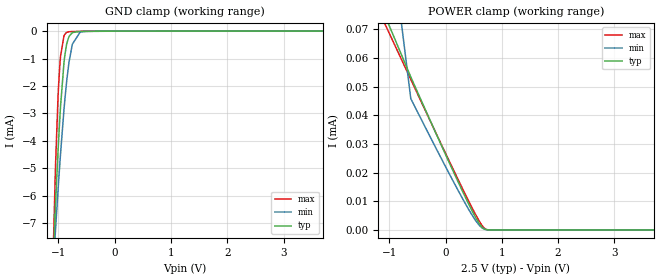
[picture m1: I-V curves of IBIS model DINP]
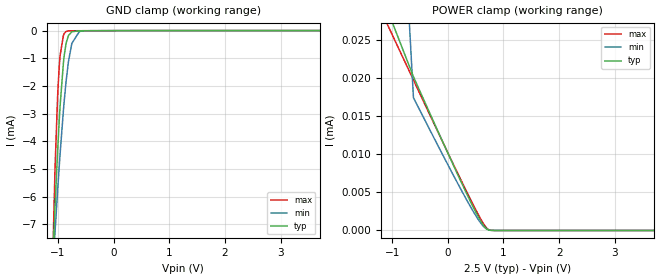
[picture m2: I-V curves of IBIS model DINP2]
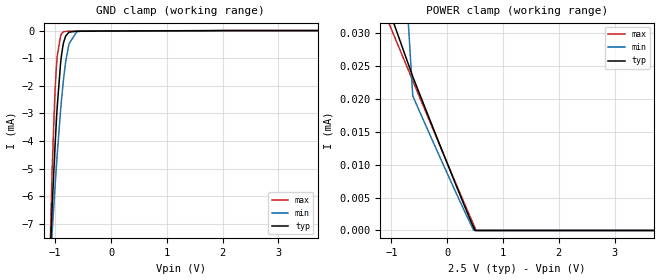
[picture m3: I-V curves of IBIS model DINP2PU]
| Texas Instruments Incorporated
| Wideband Frequency Multiplier/Buffer/Divider
| Marketing part#   Voltage Range   Package-type   #pins/pkg drawing
| LMX1906PAP   2.4V - 2.6V   HTQFP   64
[IBIS Ver]   4.1
[File name]   lmx1906.ibs
[File Rev]   1.0
[Date]   12/15/2023
[Source]   Model built from spectre simulations at:
   Texas Instruments Incorporated.
   Analog-eLab, HPA
   12500 TI Blvd
   Dallas, TX -75243
   For Support e-mail: elab_ibis@list.ti.com
[Notes]   Revision History
   Rev 1.0: 12/15/2023
   | - Initial version of the model
		| - Model generated from simulations in TISPICE/SPECTRE
		| - C_comp although listed in numerical order of value are
		| obtained from varying PVT conditions. For PVT conditions for
		| each specific value refer the buffer description under
		| respective [Model]. IBIS model user is responsible for using
		| appropriate C_comp to simulate for Signal Integrity.
		| - Warnings regarding combined Non-monotonicity of various models have been
		| reviewed and considered minor and can be ignored.
[Disclaimer]  This model is designed as an aid for customers of Texas Instruments
 TI and its licensors and suppliers make no warranties, either expressed
 or implied, with respect to this  model, including the warranties of
 merchantability or fitness for a particular purpose.
 The model is provided solely on an "as is" basis. The entire risk as to
 its quality and performance is with the customer.
[Copyright] (C)Copyright 2022 Texas Instruments Incorporated.
   All rights reserved.
[Component]   LMX1906PAP
[Manufacturer]  Texas Instruments Incorporated
[Package]   | 64 HTQFP package
|   typ   min   max
R_pkg   0.1725   0.1129   0.2855
L_pkg   2.714n   2.2186n   3.5183n
C_pkg   0.361p   0.314p   0.430p
[Pin]   signal_name   model_name   R_pin   L_pin   C_pin
1		MUXOUT			MUXOUT   0.2855	3.3842n	0.3415p
2		CE   DINP2PU   0.2536	3.3372n	0.3506p
3		SYSREFREQ_P		SYSREFREQ			0.1427	2.5185n	0.4062p
4		SYSREFREQ_N		SYSREFREQ			0.1446	2.4677n	0.4029p
5		VCC_CLKIN		POWER   0.1444	2.4377n	0.4011p
6		GND   GND   0.1465	2.5401n	0.4093p
7		CLKIN_P			CLKIN   0.1378	2.5513n	0.3934p
8		CLKIN_N			CLKIN   0.1335	2.5574n	0.3858p
9		GND   GND   0.1276	2.5225n	0.3644p
10		PWRSEL0			DINP2   0.2286	3.1682n	0.3091p
11		PWRSEL1			DINP2   0.2255	3.1183n	0.3252p
12		PWRSEL2			DINP2   0.2354	3.0653n	0.3145p
13		NC   NC   NA		NA		0.1876p
14		SCK   DINP   0.2413	3.2102n	0.3359p
15		SDI   DINP   0.2507	3.3356n	0.3545p
16		CSB   DINP   0.2811	3.4095n	0.3313p
17		CAL   DINP2PD   0.2609	3.2904n	0.3177p
18		SYSREFOUT0_N	SYSREFOUT			0.1338	2.4339n	0.4106p
19		SYSREFOUT0_P	SYSREFOUT			0.1337	2.346n	0.4077p
20		VCC01			POWER   0.125	2.3265n	0.3695p
21		GND   GND   0.1219	2.3195n	0.3653p
22		CLKOUT0_N		CLKOUT   0.1183	2.2631n	0.3573p
23		CLKOUT0_P		CLKOUT   0.1158	2.2412n	0.3551p
24		GND   GND   0.1129	2.2186n	0.3405p
25		CLK0_EN			DINP2PU   0.2001	2.7673n	0.2962p
26		CLK1_EN			DINP2PU   0.2022	2.7921n	0.2955p
27		VCC01			POWER   0.1158	2.2646n	0.3559p
28		GND   GND   0.1214	2.3129n	0.3748p
29		CLKOUT1_N		CLKOUT   0.1258	2.3939n	0.3804p
30		CLKOUT1_P		CLKOUT   0.13	2.4419n	0.3917p
31		GND   GND   0.1391	2.5338n	0.4304p
32		VBIAS01			NC   0.1511	2.6436n	0.3713p
33		SYSREFOUT1_N	SYSREFOUT			0.1629	2.6698n	0.3981p
34		SYSREFOUT1_P	SYSREFOUT			0.1536	2.6121n	0.4289p
35		DIVSEL2			DINP2   0.2536	3.4411n	0.3494p
36		DIVSEL1			DINP2   0.2393	3.3209n	0.3437p
37		DIVSEL0			DINP2   0.23	3.2291n	0.3392p
38		LOGISYSREFOUT_N	LOGICOUT			0.2284	3.2104n	0.3111p
39		LOGISYSREFOUT_P	LOGICOUT			0.2274	3.1382n	0.3282p
40		VCC_LOGICLK		POWER   0.1269	2.4538n	0.3782p
41		GND   GND   0.133	2.3535n	0.3903p
42		LOGICLKOUT_N	LOGICOUT			0.2374	2.9999n	0.3282p
43		LOGICLKOUT_P	LOGICOUT			0.2299	3.1823n	0.3066p
44		LOGIC_EN		DINP2PU   0.2321	3.2611n	0.3316p
45		MUXSEL1			DINP2   0.2423	3.3821n	0.3494p
46		MUXSEL0			DINP2   0.2574	3.5183n	0.3459p
47		SYSREFOUT2_N	SYSREFOUT			0.1535	2.6397n	0.4253p
48		SYSREFOUT2_P	SYSREFOUT			0.1637	2.6631n	0.4082p
49		VBIAS23			NC   0.1492	2.6652n	0.3821p
50		GND   GND   0.1387	2.5423n	0.4206p
51		CLKOUT2_N		CLKOUT   0.1303	2.4448n	0.3945p
52		CLKOUT2_P		CLKOUT   0.1259	2.395n	0.3887p
53		GND   GND   0.1217	2.315n	0.3737p
54		VCC23			POWER   0.116	2.2652n	0.373p
55		CLK2_EN			DINP2PU   0.2023	2.7925n	0.3032p
56		CLK3_EN			DINP2PU   0.2001	2.768n	0.2971p
57		GND   GND   0.1129	2.2196n	0.3488p
58		CLKOUT3_N		CLKOUT   0.1161	2.2426n	0.3563p
59		CLKOUT3_P		CLKOUT   0.1182	2.2641n	0.3735p
60		GND   GND   0.1225	2.3228n	0.3619p
61		VCC23			POWER   0.1255	2.3319n	0.3762p
62		SYSREFOUT3_N	SYSREFOUT			0.1341	2.3637n	0.4173p
63		SYSREFOUT3_P	SYSREFOUT			0.1341	2.441n	0.421p
64		SYSREF_EN		DINP2PU   0.2593	3.3219n	0.3135p
[Diff pin]  inv_pin  vdiff  tdelay_typ  tdelay_min  tdelay_max
  3   4   NA   NA   NA   NA
  7   8   NA   NA   NA   NA
 19   18   NA   0.0s   0.0s   0.0s
 23   22   NA   0.0s   0.0s   0.0s
 30   29   NA   0.0s   0.0s   0.0s
 34   33   NA   0.0s   0.0s   0.0s
 39   38   NA   0.0s   0.0s   0.0s
 43   42   NA   0.0s   0.0s   0.0s
 48   47   NA   0.0s   0.0s   0.0s
 52   51   NA   0.0s   0.0s   0.0s
 59   58   NA   0.0s   0.0s   0.0s
 63   62   NA   0.0s   0.0s   0.0s
| Models and submodels in the file (10): DINP (Input), DINP2 (Input), DINP2PU (Input), DINP2PD (Input), MUXOUT (Output), CLKIN (Input), SYSREFREQ (Input), CLKOUT (Output), SYSREFOUT (Output), LOGICOUT (Output)
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|   Model DINP
[Model]   DINP
Model_type   Input
Vinl = 0.4
Vinh = 1.4
|   typ   min   max
C_comp   0.0195pF   0.0186pF   0.0315pF
[Voltage Range]   2.5   2.4   2.6
[Temperature Range]   27   105   -40
[Power Clamp Reference]   2.5   2.4   2.6
[GND Clamp Reference]   0   0   0
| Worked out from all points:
|   GND clamp passes 1 mA (typ) near -0.89 V on its own axis
|   POWER clamp passes 1 mA (typ) near -1.77 V on its own axis
[GND Clamp]
|   Voltage   I(typ)   I(min)   I(max)
-2.5V     -99.67mA   -67.42mA   -181.3mA
-1.113V   -9.277mA   -9.317mA   -9.589mA
-1.052V   -6.327mA   -7.259mA   -4.916mA
-1.008V   -4.376mA   -5.809mA   -2.402mA
-977.5mV  -3.241mA   -4.898mA   -1.299mA
-962.5mV  -2.733mA   -4.463mA   -914.2uA
-902.5mV  -1.168mA   -2.88mA    -182.1uA
-850mV    -435.4uA   -1.755mA   -43.32uA
-812.5mV  -195.5uA   -1.133mA   -23.19uA
-752.5mV  -53.81uA   -476.9uA   -16.37uA
-572.5mV  -11.42uA   -23.03uA   -8.659uA
5V        0A         0A         0A
[POWER Clamp]
|   Voltage   I(typ)   I(min)   I(max)
-2.5V     13.01mA    14.14mA    11.88mA
-1.337V   87.06uA    159.9uA    82.89uA
-617.5mV  53.41uA    45.83uA    52.55uA
-47.5mV   28.4uA     23.9uA     28.74uA
327.5mV   12.45uA    10.06uA    13.4uA
545mV     3.985uA    2.992uA    4.984uA
605mV     2.064uA    1.51uA     2.9uA
680mV     464.7nA    375.9nA    816.5nA
725mV     113.8nA    119.2nA    188.1nA
807.5mV   4.801nA    11.39nA    3.57nA
5V        0A         0A         0A
|   Model DINP2
[Model]   DINP2
Model_type   Input
Vinl = 0.4
Vinh = 1.4
|   typ   min   max
C_comp   0.0195pF   0.0186pF   0.0315pF
[Voltage Range]   2.5   2.4   2.6
[Temperature Range]   27   105   -40
[Power Clamp Reference]   2.5   2.4   2.6
[GND Clamp Reference]   0   0   0
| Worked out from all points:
|   GND clamp passes 1 mA (typ) near -0.89 V on its own axis
|   POWER clamp passes 1 mA (typ) near -1.77 V on its own axis
[GND Clamp]
|   Voltage   I(typ)   I(min)   I(max)
-2.5V     -99.57mA   -67.32mA   -181.2mA
-1.113V   -9.249mA   -9.291mA   -9.563mA
-1.052V   -6.302mA   -7.235mA   -4.893mA
-1.008V   -4.352mA   -5.787mA   -2.381mA
-977.5mV  -3.219mA   -4.877mA   -1.279mA
-962.5mV  -2.712mA   -4.442mA   -895.3uA
-902.5mV  -1.15mA    -2.862mA   -166uA
-850mV    -419.4uA   -1.739mA   -29.61uA
-812.5mV  -181.2uA   -1.118mA   -11.15uA
-752.5mV  -42.15uA   -464.8uA   -6.933uA
-572.5mV  -6.468uA   -16.88uA   -5.399uA
5V        0A         0A         0A
[POWER Clamp]
|   Voltage   I(typ)   I(min)   I(max)
-2.5V     12.92mA    14.06mA    11.79mA
-1.337V   33.75uA    113.8uA    31.04uA
-617.5mV  20.23uA    17.47uA    19.79uA
-40mV     10.83uA    9.222uA    10.85uA
350mV     4.672uA    3.871uA    4.935uA
560mV     1.625uA    1.3uA      1.921uA
642.5mV   650.5nA    526.3nA    873.5nA
702.5mV   190.6nA    176.9nA    287.2nA
755mV     36.65nA    47.43nA    46.65nA
830mV     1.587nA    4.923nA    736.5pA
5V        0A         0A         0A
|   Model DINP2PU
[Model]   DINP2PU
Model_type   Input
Vinl = 0.4
Vinh = 1.4
|   typ   min   max
C_comp   0.0195pF   0.0186pF   0.0315pF
[Voltage Range]   2.5   2.4   2.6
[Temperature Range]   27   105   -40
[Power Clamp Reference]   2.5   2.4   2.6
[GND Clamp Reference]   0   0   0
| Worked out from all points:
|   GND clamp passes 1 mA (typ) near -0.89 V on its own axis
|   POWER clamp passes 1 mA (typ) near -1.77 V on its own axis
[GND Clamp]
|   Voltage   I(typ)   I(min)   I(max)
-2.5V     -99.59mA   -67.35mA   -181.2mA
-1.113V   -9.267mA   -9.307mA   -9.58mA
-1.052V   -6.32mA    -7.251mA   -4.911mA
-1.008V   -4.37mA    -5.803mA   -2.398mA
-977.5mV  -3.237mA   -4.893mA   -1.296mA
-962.5mV  -2.73mA    -4.458mA   -912.3uA
-902.5mV  -1.167mA   -2.878mA   -182.8uA
-850mV    -436.3uA   -1.755mA   -46.1uA
-812.5mV  -197.9uA   -1.134mA   -27.46uA
-752.5mV  -58.61uA   -479.8uA   -22.96uA
-572.5mV  -22.02uA   -31.03uA   -20.56uA
5V        0A         0A         0A
[POWER Clamp]
|   Voltage   I(typ)   I(min)   I(max)
-2.5V     12.93mA    14.07mA    11.81mA
-1.337V   40.52uA    120.1uA    37.43uA
-617.5mV  23.35uA    20.41uA    22.74uA
162.5mV   6.774uA    5.627uA    6.978uA
425mV     1.389uA    878.5nA    1.8uA
470mV     499.3nA    103.7nA    934nA
485mV     207nA      0A         647.8nA
492.5mV   61.71nA    0A         505.2nA
515mV     0A         0A         80.2nA
530mV     0A         0A         0A
5V        0A         0A         0A
